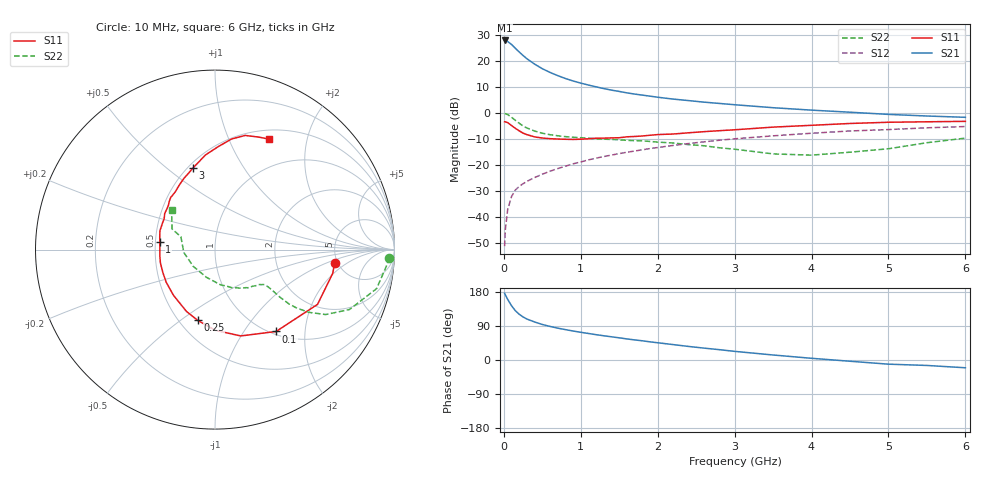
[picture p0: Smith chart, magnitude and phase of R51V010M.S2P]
! SIEMENS Small Signal Semiconductors
! BFR183
! Si NPN RF Bipolar Junction Transistor in SOT23
! VCE = 1 V  IC = 10 mA
! Common Emitter S-Parameters:  May  1996
# GHz  S  MA  R  50
!  f  S11  S21  S12  S22
! GHz  MAG  ANG  MAG  ANG  MAG  ANG  MAG  ANG
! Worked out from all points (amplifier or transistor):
!   36 points, 10 MHz to 6 GHz, reference 50 ohm
!   highest |S21| = 27.9 dB at 10 MHz (marker M1)
!   |S21| within 3 dB of that: start of sweep to 148.9 MHz
!   unconditionally stable (mu >= 1): 692.9 MHz to 2.701 GHz
!   at 250 MHz: K = 0.65, MSG = 24.7 dB, |S12| = -27.3 dB
!   at 1.4 GHz: K = 1.07, MAG = 10.9 dB, |S12| = -16.3 dB
!   at 6 GHz: K = 0.93, MSG = 1.8 dB, |S12| = -5.3 dB
!   S11 on the Smith chart (normalised r, x): 10 MHz: 4.73, -1.25; 100 MHz: 1.05, -1.42; 250 MHz: 0.62, -0.58; 1 GHz: 0.53, +0.05; 3 GHz: 0.53, +0.62; 6 GHz: 0.61, +1.42
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0.01  0.6708 -6.2  24.75 176.0  0.0027 90.1  0.9725 -2.7
0.02  0.6692 -11.4  24.55 171.6  0.0057 85.2  0.959 -5.6
0.05  0.6477 -28.1  23.59 159.9  0.0137 78.2  0.9261 -13.6
0.1  0.5691 -53.3  20.73 143.2  0.0244 67.9  0.8205 -24.0
0.15  0.5019 -73.4  17.46 130.0  0.0326 63.1  0.7151 -30.4
0.2  0.4496 -89.8  14.84 120.7  0.0382 60.9  0.6282 -33.8
0.25  0.4059 -103.7  12.69 113.6  0.0431 59.9  0.5579 -35.6
0.3  0.3797 -114.7  11 108.1  0.0478 59.8  0.5102 -36.3
0.4  0.3436 -132.5  8.67 100.3  0.0566 60.4  0.4462 -36.2
0.5  0.3268 -146.5  7.072 93.7  0.0657 61.6  0.4043 -35.6
0.6  0.3173 -156.5  6.003 88.6  0.075 62.4  0.3787 -35.2
0.7  0.3131 -166.4  5.208 84.1  0.0842 62.9  0.3613 -35.1
0.8  0.3092 -173.7  4.582 80.2  0.0937 62.9  0.3479 -35.1
1  0.31 172.5  3.731 73.1  0.1132 63.2  0.3313 -35.9
1.1  0.3159 167.1  3.425 70.0  0.124 63.1  0.324 -37.1
1.6  0.345 144.3  2.422 55.6  0.174 59.7  0.2949 -43.6
2.2  0.3904 124.6  1.838 40.7  0.2352 54.1  0.2622 -55.4
3  0.4709 105.1  1.431 22.8  0.3157 44.4  0.1992 -80.8
3.5  0.5303 95.7  1.254 13.2  0.3602 37.7  0.1616 -107.1
4.5  0.6231 81.5  1.027 -3.3  0.4468 24.7  0.1744 -174.6
5.5  0.6716 69.1  0.868 -14.4  0.5139 12.8  0.2656 154.3
6  0.685 64.0  0.819 -20.5  0.5445 5.2  0.3254 137.9
